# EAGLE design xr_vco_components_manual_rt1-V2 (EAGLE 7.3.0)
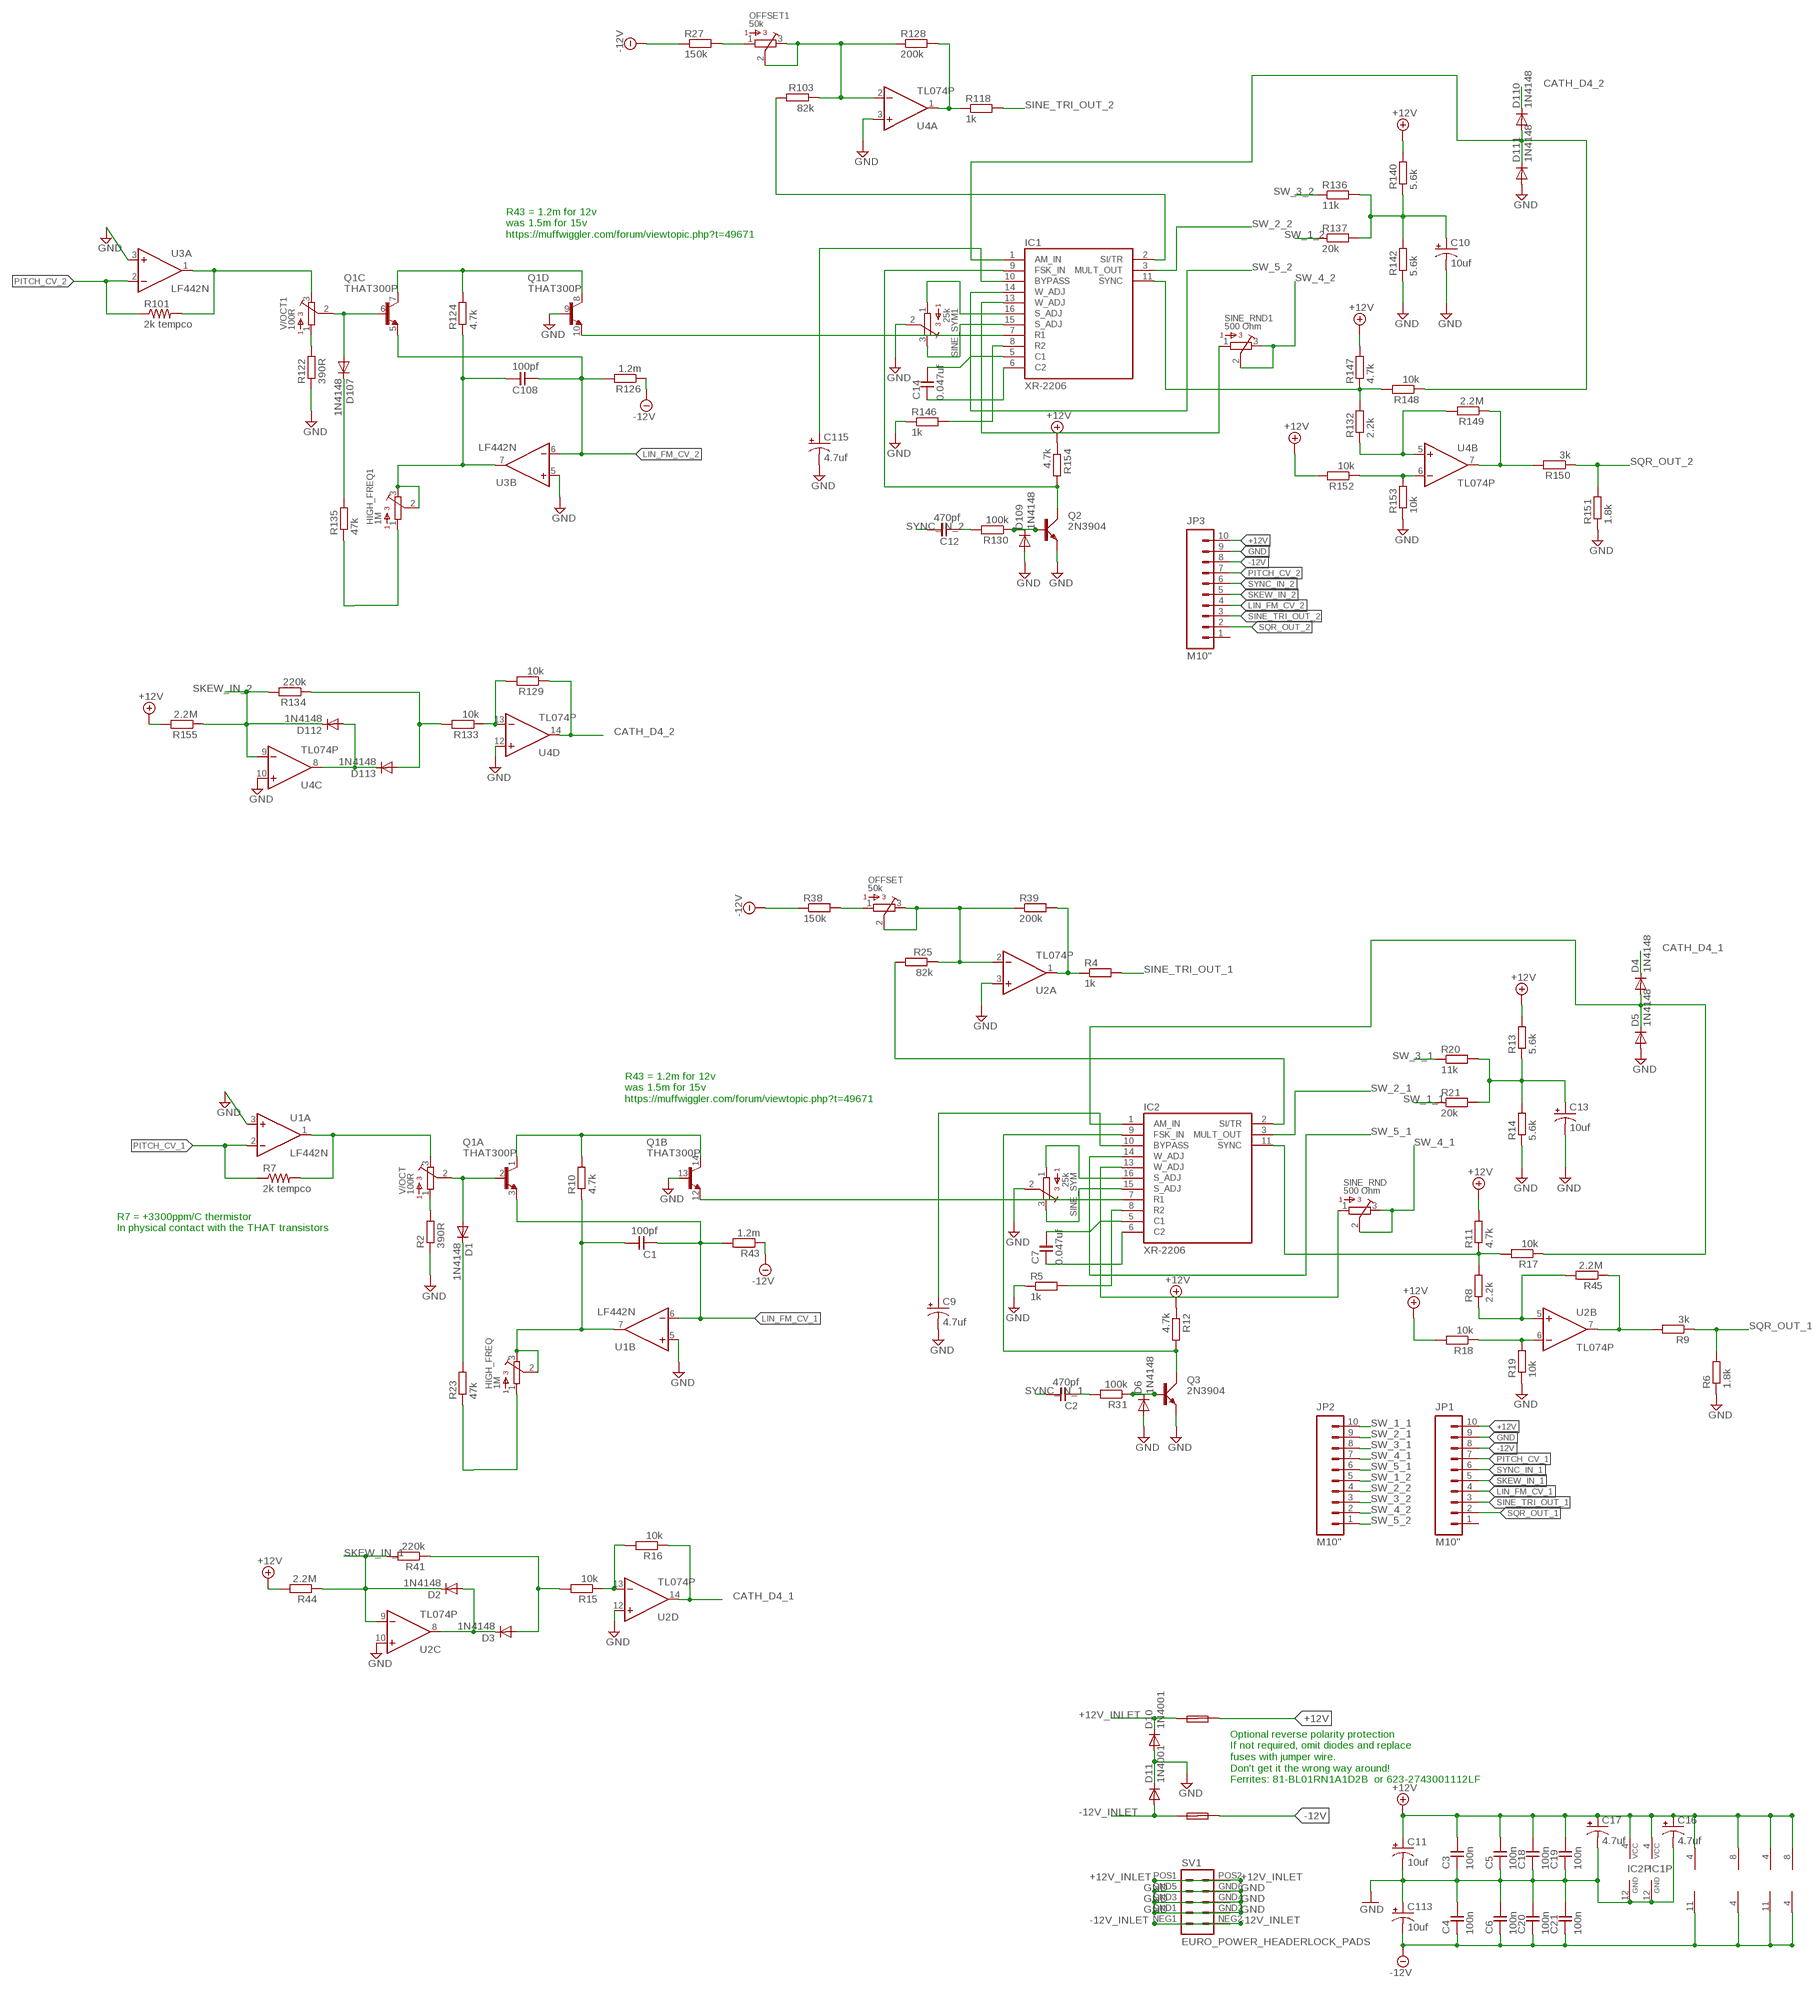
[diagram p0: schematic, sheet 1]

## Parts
C1  100pf  C-EU050-024X044  [C050-024X044]
C2  470pf  C-EU050-024X044  [C050-024X044]
C3  100n  C-EU050-024X044  [C050-024X044]
C4  100n  C-EU050-024X044  [C050-024X044]
C5  100n  C-EU050-024X044  [C050-024X044]
C6  100n  C-EU050-024X044  [C050-024X044]
C7  0.047uf  C-EU050-024X044  [C050-024X044]
C9  4.7uf  CAP_POLPTH2  [CPOL-RADIAL-10UF-25V]
C10  10uf  CAP_POLPTH2  [CPOL-RADIAL-10UF-25V]
C11  10uf  CAP_POLPTH2  [CPOL-RADIAL-10UF-25V]
C12  470pf  C-EU050-024X044  [C050-024X044]
C13  10uf  CAP_POLPTH2  [CPOL-RADIAL-10UF-25V]
C14  0.047uf  C-EU050-024X044  [C050-024X044]
C16  4.7uf  CAP_POLPTH2  [CPOL-RADIAL-10UF-25V]
C17  4.7uf  CAP_POLPTH2  [CPOL-RADIAL-10UF-25V]
C18  100n  C-EU050-024X044  [C050-024X044]
C19  100n  C-EU050-024X044  [C050-024X044]
C20  100n  C-EU050-024X044  [C050-024X044]
C21  100n  C-EU050-024X044  [C050-024X044]
C108  100pf  C-EU050-024X044  [C050-024X044]
C113  10uf  CAP_POLPTH2  [CPOL-RADIAL-10UF-25V]
C115  4.7uf  CAP_POLPTH2  [CPOL-RADIAL-10UF-25V]
D1  1N4148  SMALL_DIODEDO35-7  [DO35-7]
D2  1N4148  SMALL_DIODEDO35-7  [DO35-7]
D3  1N4148  SMALL_DIODEDO35-7  [DO35-7]
D4  1N4148  SMALL_DIODEDO35-7  [DO35-7]
D5  1N4148  SMALL_DIODEDO35-7  [DO35-7]
D6  1N4148  SMALL_DIODEDO35-7  [DO35-7]
D10  1N4001  1N4004  [DO41-10]
D11  1N4001  1N4004  [DO41-10]
D107  1N4148  SMALL_DIODEDO35-7  [DO35-7]
D109  1N4148  SMALL_DIODEDO35-7  [DO35-7]
D110  1N4148  SMALL_DIODEDO35-7  [DO35-7]
D111  1N4148  SMALL_DIODEDO35-7  [DO35-7]
D112  1N4148  SMALL_DIODEDO35-7  [DO35-7]
D113  1N4148  SMALL_DIODEDO35-7  [DO35-7]
F1  FUSE  PTC_FUSEPOLY_FUSE  [C050H075X075]
F2  FUSE  PTC_FUSEPOLY_FUSE  [C050H075X075]
HIGH_FREQ  1M  BOURNS_3362P_TRIMMERP  [BOURNS_3362P_TRIMMER]
HIGH_FREQ1  1M  BOURNS_3362P_TRIMMERP  [BOURNS_3362P_TRIMMER]
IC1  XR-2206  [DIL16]
IC2  XR-2206  [DIL16]
JP1  M10"  [1X10]
JP2  M10"  [1X10]
JP3  M10"  [1X10]
OFFSET  50k  BOURNS_3362P_TRIMMERP  [BOURNS_3362P_TRIMMER]
OFFSET1  50k  BOURNS_3362P_TRIMMERP  [BOURNS_3362P_TRIMMER]
Q1  THAT300P  [DIL14]
Q2  2N3904  [TO92D]
Q3  2N3904  [TO92D]
R2  390R  RESISTOR7MM  [7MM_RESISTOR]
R4  1k  RESISTOR7MM  [7MM_RESISTOR]
R5  1k  RESISTOR7MM  [7MM_RESISTOR]
R6  1.8k  RESISTOR7MM  [7MM_RESISTOR]
R7  2k tempco  R-US_0309/12  [0309/12]
R8  2.2k  RESISTOR7MM  [7MM_RESISTOR]
R9  3k  RESISTOR7MM  [7MM_RESISTOR]
R10  4.7k  RESISTOR7MM  [7MM_RESISTOR]
R11  4.7k  RESISTOR7MM  [7MM_RESISTOR]
R12  4.7k  RESISTOR7MM  [7MM_RESISTOR]
R13  5.6k  RESISTOR7MM  [7MM_RESISTOR]
R14  5.6k  RESISTOR7MM  [7MM_RESISTOR]
R15  10k  RESISTOR7MM  [7MM_RESISTOR]
R16  10k  RESISTOR7MM  [7MM_RESISTOR]
R17  10k  RESISTOR7MM  [7MM_RESISTOR]
R18  10k  RESISTOR7MM  [7MM_RESISTOR]
R19  10k  RESISTOR7MM  [7MM_RESISTOR]
R20  11k  RESISTOR7MM  [7MM_RESISTOR]
R21  20k  RESISTOR7MM  [7MM_RESISTOR]
R23  47k  RESISTOR7MM  [7MM_RESISTOR]
R25  82k  RESISTOR7MM  [7MM_RESISTOR]
R27  150k  RESISTOR7MM  [7MM_RESISTOR]
R31  100k  RESISTOR7MM  [7MM_RESISTOR]
R38  150k  RESISTOR7MM  [7MM_RESISTOR]
R39  200k  RESISTOR7MM  [7MM_RESISTOR]
R41  220k  RESISTOR7MM  [7MM_RESISTOR]
R43  1.2m  RESISTOR7MM  [7MM_RESISTOR]
R44  2.2M  RESISTOR7MM  [7MM_RESISTOR]
R45  2.2M  RESISTOR7MM  [7MM_RESISTOR]
R101  2k tempco  R-US_0309/12  [0309/12]
R103  82k  RESISTOR7MM  [7MM_RESISTOR]
R118  1k  RESISTOR7MM  [7MM_RESISTOR]
R122  390R  RESISTOR7MM  [7MM_RESISTOR]
R124  4.7k  RESISTOR7MM  [7MM_RESISTOR]
R126  1.2m  RESISTOR7MM  [7MM_RESISTOR]
R128  200k  RESISTOR7MM  [7MM_RESISTOR]
R129  10k  RESISTOR7MM  [7MM_RESISTOR]
R130  100k  RESISTOR7MM  [7MM_RESISTOR]
R132  2.2k  RESISTOR7MM  [7MM_RESISTOR]
R133  10k  RESISTOR7MM  [7MM_RESISTOR]
R134  220k  RESISTOR7MM  [7MM_RESISTOR]
R135  47k  RESISTOR7MM  [7MM_RESISTOR]
R136  11k  RESISTOR7MM  [7MM_RESISTOR]
R137  20k  RESISTOR7MM  [7MM_RESISTOR]
R140  5.6k  RESISTOR7MM  [7MM_RESISTOR]
R142  5.6k  RESISTOR7MM  [7MM_RESISTOR]
R146  1k  RESISTOR7MM  [7MM_RESISTOR]
R147  4.7k  RESISTOR7MM  [7MM_RESISTOR]
R148  10k  RESISTOR7MM  [7MM_RESISTOR]
R149  2.2M  RESISTOR7MM  [7MM_RESISTOR]
R150  3k  RESISTOR7MM  [7MM_RESISTOR]
R151  1.8k  RESISTOR7MM  [7MM_RESISTOR]
R152  10k  RESISTOR7MM  [7MM_RESISTOR]
R153  10k  RESISTOR7MM  [7MM_RESISTOR]
R154  4.7k  RESISTOR7MM  [7MM_RESISTOR]
R155  2.2M  RESISTOR7MM  [7MM_RESISTOR]
SINE_RND  500 Ohm  BOURNS_3362P_TRIMMERP  [BOURNS_3362P_TRIMMER]
SINE_RND1  500 Ohm  BOURNS_3362P_TRIMMERP  [BOURNS_3362P_TRIMMER]
SINE_SYM  25k  BOURNS_3362P_TRIMMERP  [BOURNS_3362P_TRIMMER]
SINE_SYM1  25k  BOURNS_3362P_TRIMMERP  [BOURNS_3362P_TRIMMER]
SV1  EURO_POWER_HEADERLOCK_PADS  [EURO_PWR_HEADER_LOCK]
U1  LF442N  [DIL08]
U2  TL074P  [DIL14]
U3  LF442N  [DIL08]
U4  TL074P  [DIL14]
V/OCT  100R  BOURNS_3362P_TRIMMERP  [BOURNS_3362P_TRIMMER]
V/OCT1  100R  BOURNS_3362P_TRIMMERP  [BOURNS_3362P_TRIMMER]

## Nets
+12V: C3.1 C5.1 C11.1(+) C16.1(+) C17.1(+) C18.1 C19.1 F1.2 IC1.4(VCC) IC2.4(VCC) JP1.10 JP3.10 R11.2 R12.1 R13.2 R18.2 R44.2 R140.2 R147.2 R152.2 R154.1 R155.2 U1.8(P:V+) U2.4(P:V+) U3.8(P:V+) U4.4(P:V+)
+12V_INLET [power]: D10.C F1.1 SV1.POS1 SV1.POS2
-12V: C4.2 C6.2 C20.2 C21.2 C113.2(-) F2.2 JP1.8 JP3.8 R27.1 R38.1 R43.1 R126.1 U1.4(P:V-) U2.11(P:V-) U3.4(P:V-) U4.11(P:V-)
-12V_INLET [power]: D11.A F2.1 SV1.NEG1 SV1.NEG2
CATH_D4_1: D4.C R16.1 U2.14(D:OUT)
CATH_D4_2: D110.C R129.1 U4.14(D:OUT)
GND: C3.2 C4.1 C5.2 C6.1 C9.2(-) C10.2(-) C11.2(-) C13.2(-) C16.2(-) C17.2(-) C18.2 C19.2 C20.1 C21.1 C113.1(+) C115.2(-) D5.A D6.A D10.A D11.C D109.A D111.A IC1.12(GND) IC2.12(GND) JP1.9 JP3.9 Q1.9(D:B) Q1.13(B:B) Q2.E Q3.E R2.1 R5.1 R6.1 R14.1 R19.1 R122.1 R142.1 R146.1 R151.1 R153.1 SINE_SYM1.2 SINE_SYM.2 SV1.GND1 SV1.GND2 SV1.GND3 SV1.GND4 SV1.GND5 SV1.GND6 U1.3(A:+IN) U1.5(B:+IN) U2.3(A:+IN) U2.10(C:+IN) U2.12(D:+IN) U3.3(A:+IN) U3.5(B:+IN) U4.3(A:+IN) U4.10(C:+IN) U4.12(D:+IN)
LIN_FM_CV_1: C1.2 JP1.4 Q1.3(A:E) R43.2 U1.6(B:-IN)
LIN_FM_CV_2: C108.2 JP3.4 Q1.5(C:E) R126.2 U3.6(B:-IN)
N$1: IC2.7(R1) Q1.12(B:E)
N$2: D1.C R23.2
N$3: HIGH_FREQ.1 R23.1
N$4: R101.2 U3.1(A:OUT) V/OCT1.3
N$5: IC2.2(SI/TR) R25.2
N$6: R122.2 V/OCT1.1
N$7: R7.2 U1.1(A:OUT) V/OCT.3
N$8: OFFSET.2 OFFSET.3 R25.1 R39.1 U2.2(A:-IN)
N$9: R2.2 V/OCT.1
N$10: D1.A Q1.2(A:B) V/OCT.2
N$11: Q1.1(A:C) Q1.14(B:C) R10.2
N$12: OFFSET.1 R38.2
N$13: R4.1 R39.2 U2.1(A:OUT)
N$14: D107.A Q1.6(C:B) V/OCT1.2
N$15: C1.1 HIGH_FREQ.2 HIGH_FREQ.3 R10.1 U1.7(B:OUT)
N$16: C13.1(+) R13.1 R14.2 R20.2 R21.2
N$17: IC2.16(S_ADJ) SINE_SYM.1
N$18: Q1.7(C:C) Q1.8(D:C) R124.2
N$19: C108.1 HIGH_FREQ1.2 HIGH_FREQ1.3 R124.1 U3.7(B:OUT)
N$20: IC2.13(W_ADJ) SINE_RND.1
N$21: IC2.15(S_ADJ) SINE_SYM.3
N$22: IC2.8(R2) R5.2
N$23: R18.1 R19.2 U2.6(B:-IN)
N$24: R9.2 R45.1 U2.7(B:OUT)
N$25: R15.1 R16.2 U2.13(D:-IN)
N$26: R8.1 R45.2 U2.5(B:+IN)
N$27: D4.A D5.C IC2.1(AM_IN) R17.1
N$28: C2.2 R31.2
N$29: D6.C Q3.B R31.1
N$30: IC2.11(SYNC) R8.2 R11.1 R17.2
N$31: IC2.9(FSK_IN) Q3.C R12.2
N$32: C7.2 IC2.6(C2)
N$33: C7.1 IC2.5(C1)
N$34: C9.1(+) IC2.10(BYPASS)
N$35: D2.A D3.C U2.8(C:OUT)
N$36: D3.A R15.2 R41.1
N$37: IC1.7(R1) Q1.10(D:E)
N$38: HIGH_FREQ1.1 R135.1
N$39: D107.C R135.2
N$40: IC1.2(SI/TR) R103.2
N$41: OFFSET1.2 OFFSET1.3 R103.1 R128.1 U4.2(A:-IN)
N$42: OFFSET1.1 R27.2
N$43: R118.1 R128.2 U4.1(A:OUT)
N$44: C10.1(+) R136.2 R137.2 R140.1 R142.2
N$45: IC1.13(W_ADJ) SINE_RND1.1
N$46: IC1.16(S_ADJ) SINE_SYM1.1
N$47: IC1.15(S_ADJ) SINE_SYM1.3
N$48: IC1.8(R2) R146.2
N$49: R152.1 R153.2 U4.6(B:-IN)
N$50: R149.1 R150.2 U4.7(B:OUT)
N$51: R132.1 R149.2 U4.5(B:+IN)
N$52: IC1.11(SYNC) R132.2 R147.1 R148.2
N$53: D110.A D111.C IC1.1(AM_IN) R148.1
N$54: C12.2 R130.2
N$55: D109.C Q2.B R130.1
N$56: IC1.9(FSK_IN) Q2.C R154.2
N$57: C14.2 IC1.6(C2)
N$58: C14.1 IC1.5(C1)
N$59: R129.2 R133.1 U4.13(D:-IN)
N$60: D112.A D113.C U4.8(C:OUT)
N$61: D113.A R133.2 R134.1
N$62: C115.1(+) IC1.10(BYPASS)
PITCH_CV_1: JP1.7 R7.1 U1.2(A:-IN)
PITCH_CV_2: JP3.7 R101.1 U3.2(A:-IN)
SINE_TRI_OUT_1: JP1.3 R4.2
SINE_TRI_OUT_2: JP3.3 R118.2
SKEW_IN_1: D2.C JP1.5 R41.2 R44.1 U2.9(C:-IN)
SKEW_IN_2: D112.C JP3.5 R134.2 R155.1 U4.9(C:-IN)
SQR_OUT_1: JP1.2 R6.2 R9.1
SQR_OUT_2: JP3.2 R150.1 R151.2
SW_1_1: JP2.10 R21.1
SW_1_2: JP2.5 R137.1
SW_2_1: IC2.3(MULT_OUT) JP2.9
SW_2_2: IC1.3(MULT_OUT) JP2.4
SW_3_1: JP2.8 R20.1
SW_3_2: JP2.3 R136.1
SW_4_1: JP2.7 SINE_RND.2 SINE_RND.3
SW_4_2: JP2.2 SINE_RND1.2 SINE_RND1.3
SW_5_1: IC2.14(W_ADJ) JP2.6
SW_5_2: IC1.14(W_ADJ) JP2.1
SYNC_IN_1: C2.1 JP1.6
SYNC_IN_2: C12.1 JP3.6
Unconnected: JP1.1 JP3.1

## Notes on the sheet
- R43 = 1.2m for 12v
  was 1.5m for 15v
  https://muffwiggler.com/forum/viewtopic.php?t=49671
- R43 = 1.2m for 12v
  was 1.5m for 15v
  https://muffwiggler.com/forum/viewtopic.php?t=49671
- R7 = +3300ppm/C thermistor
  In physical contact with the THAT transistors
- Optional reverse polarity protection
  If not required, omit diodes and replace
  fuses with jumper wire. 
  Don't get it the wrong way around! 
  Ferrites: 81-BL01RN1A1D2B  or 623-2743001112LF

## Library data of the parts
C1-C7 C12 C14 C18-C21 C108 = TomW:C-EU: CAPACITOR, European symbol
C9-C11 C13 C16 C17 C113 C115 = SparkFun-Passives:CAP_POL: Capacitor Polarized
D1-D6 D107 D109-D113 = MusicThingModular:SMALL_DIODE: Small Signal Diode
D10 D11 = diode:1N4004: DIODE
F1 F2 = TomW:PTC_FUSE
HIGH_FREQ HIGH_FREQ1 OFFSET OFFSET1 SINE_RND SINE_RND1 SINE_SYM SINE_SYM1 V/OCT V/OCT1 = MusicThingModular:BOURNS_3362P_TRIMMER: 3362 Series 1/4" Square Trimmer
IC1 IC2 = exar:XR-2206: Monolithic FUNCTION GENERATOR; OC_FARNELL: unknown; OC_NEWARK: unknown
JP1-JP3 = SparkFun-Connectors:M10: Header 10 Standard 10-pin 0.1" header. Use with straight break away headers (SKU : PRT-00116), right angle break away headers (PRT-00553), swiss pins (PRT-00743), machine pins (PRT-00117), and female headers (PRT-00115).
Q1 = that-corp:THAT300: 4-Matched NPN Transistors
Q2 Q3 = transistor-small-signal:2N3904: NPN TRANSISTOR
R2 R4-R6 R8-R21 R23 R25 R27 R31 R38 R39 R41 R43-R45 R103 R118 R122 R124 R126 R128-R130 R132-R137 R140 R142 R146-R155 = MusicThingModular:RESISTOR: Standard resistor, various versions
R7 R101 = resistor:R-US_: RESISTOR, American symbol
SV1 = MusicThingModular:EURO_POWER_HEADER: Power Header 10 pin power header for Eurorack Power Supplies Variants with fatter pads for easier soldering, and the LOCK variant which has 5mil offset pins to hold the component in place before soldering
U1 U3 = linear:LF442: OP AMP
U2 U4 = linear:TL074: OP AMP

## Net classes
1 power: width 0.406 mm
2 ground: width 0.305 mm

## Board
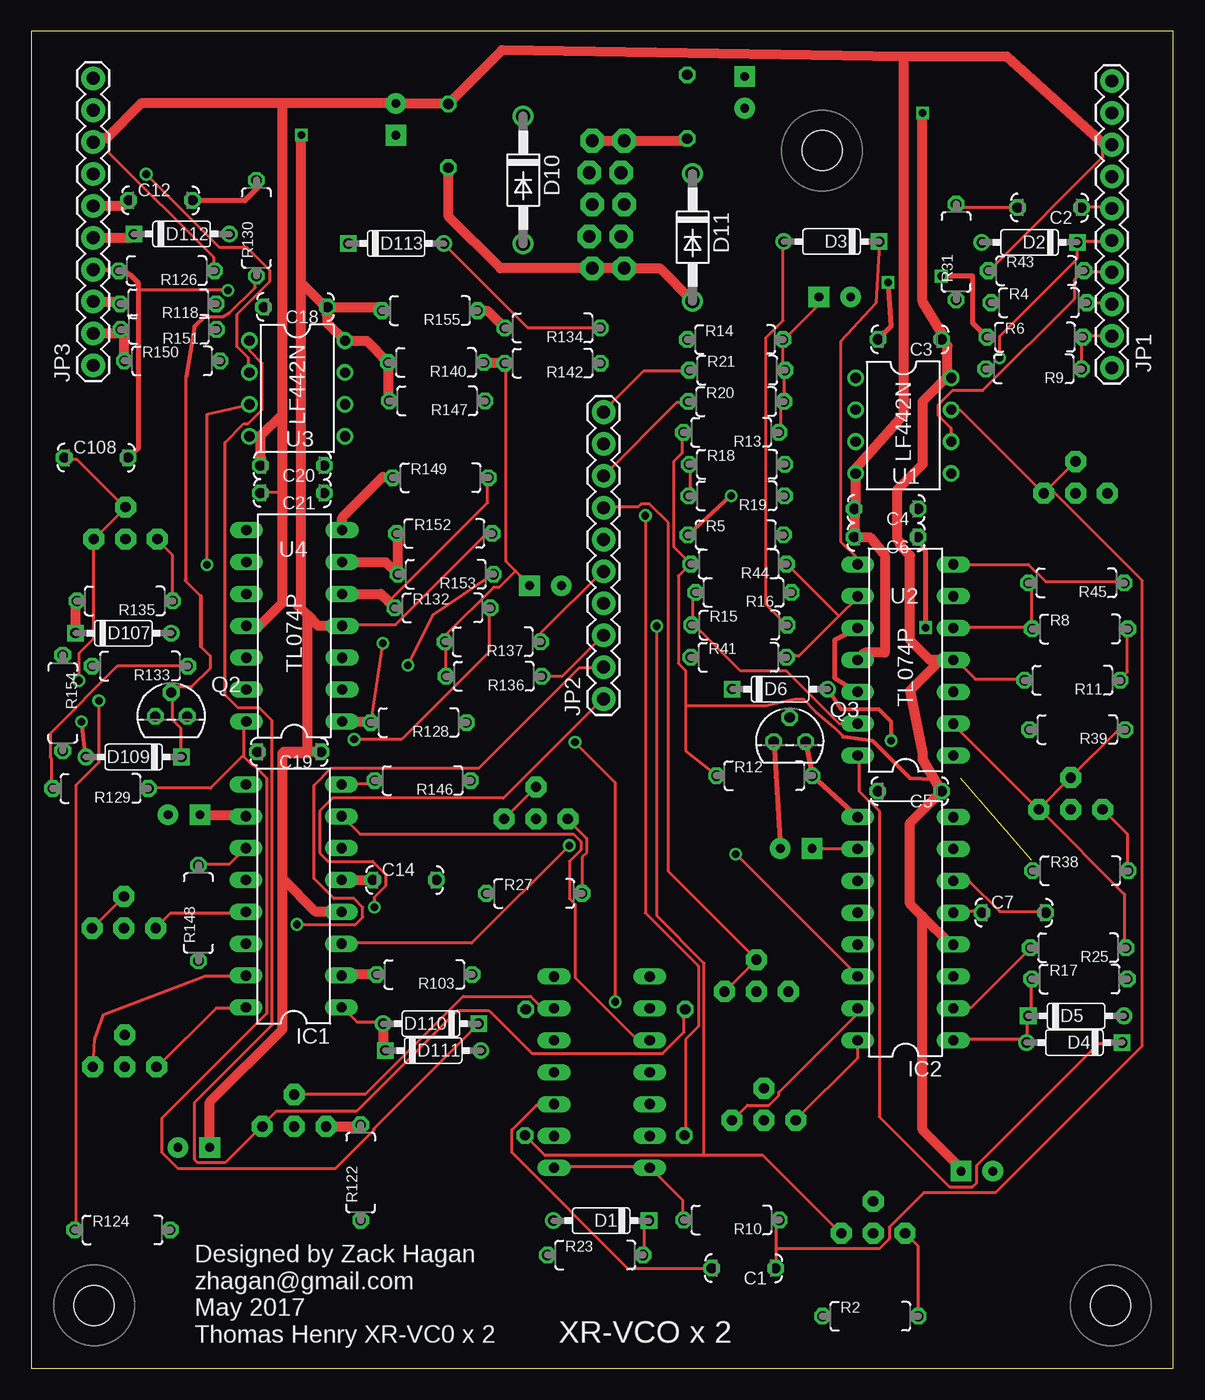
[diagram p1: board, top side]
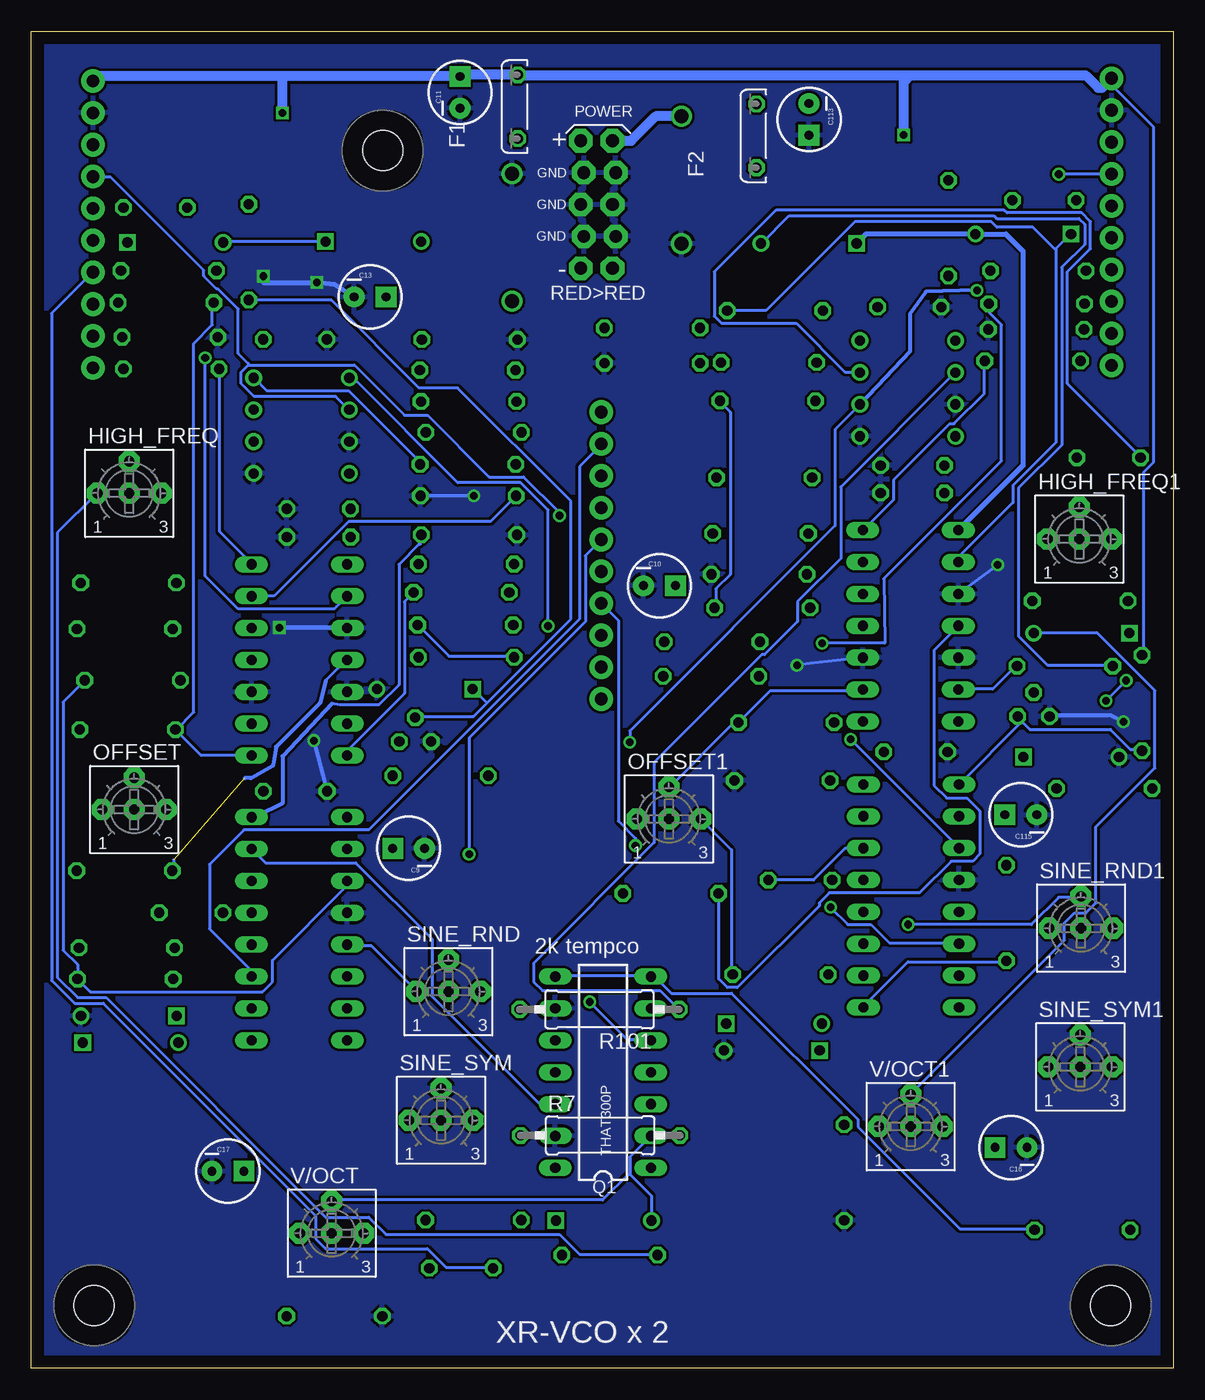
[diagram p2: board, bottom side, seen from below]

Size 91 x 106.5 mm. Coordinates in mm from the lower left corner, seen from the top.
Outline: 0,0 91,0 91,106.5 0,106.5 0,0
Copper layers (1*16): Top 0.035mm / dielectric 1.5mm / Bottom 0.035mm
Design rules "default *": minimum track width 10mil, minimum drill 19mil, track to track 8mil, track to pad 8mil, pad to pad 8mil, via to via 8mil, smd to smd 8mil, copper to edge 40mil, drill to drill 8mil, minimum pad ring 10mil, minimum via ring 8mil, stop-mask expansion 4mil, vias tented up to drill 0mil, thermal gap 10mil

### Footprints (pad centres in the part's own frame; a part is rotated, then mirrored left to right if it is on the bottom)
C050-024X044 = drill 0.813 octagon: 1 -2.54,0; 2 2.54,0
CPOL-RADIAL-10UF-25V = drill 0.7 pad 1.651 square: 1 1.27,0 | drill 0.7 pad 1.651: 2 -1.27,0
DO35-7 = drill 0.813: A 3.81,0 | drill 0.813 square: C -3.81,0
DO41-10 = drill 1.118: A 5.08,0; C -5.08,0
C050H075X075 = drill 0.813 octagon: 1 -2.54,0; 2 2.54,0
BOURNS_3362P_TRIMMER = drill 0.813 pad 1.676 octagon: 1 -2.54,0; 2 0,2.54; 3 2.54,0; 4 0,0
DIL16 = drill 0.813 long: 1 -8.89,-3.81; 2 -6.35,-3.81; 3 -3.81,-3.81; 4 -1.27,-3.81; 5 1.27,-3.81; 6 3.81,-3.81; 7 6.35,-3.81; 8 8.89,-3.81; 9 8.89,3.81; 10 6.35,3.81; 11 3.81,3.81; 12 1.27,3.81; 13 -1.27,3.81; 14 -3.81,3.81; 15 -6.35,3.81; 16 -8.89,3.81
1X10 = drill 1.016 pad 1.88: 1 0,0; 2 2.54,0; 3 5.08,0; 4 7.62,0; 5 10.16,0; 6 12.7,0; 7 15.24,0; 8 17.78,0; 9 20.32,0; 10 22.86,0
DIL14 = drill 0.813 long: 1 -7.62,-3.81; 2 -5.08,-3.81; 3 -2.54,-3.81; 4 0,-3.81; 5 2.54,-3.81; 6 5.08,-3.81; 7 7.62,-3.81; 8 7.62,3.81; 9 5.08,3.81; 10 2.54,3.81; 11 0,3.81; 12 -2.54,3.81; 13 -5.08,3.81; 14 -7.62,3.81
TO92D = drill 0.813 octagon: B 0,1.905; C 1.27,0; E -1.27,0
7MM_RESISTOR = drill 0.813 octagon: 1 -3.81,0; 2 3.81,0
0309/12 = drill 0.813 octagon: 1 -6.35,0; 2 6.35,0
EURO_PWR_HEADER_LOCK = drill 1.016 pad 1.88 octagon: GND1 -2.54,1.143; GND2 -2.54,-1.397; GND3 0,1.397; GND4 0,-1.143; GND5 2.54,1.143; GND6 2.54,-1.397; NEG1 -5.08,1.397; NEG2 -5.08,-1.143; POS1 5.08,1.397; POS2 5.08,-1.143
DIL08 = drill 0.813 pad 1.27: 1 -3.81,-3.81; 2 -1.27,-3.81; 3 1.27,-3.81; 4 3.81,-3.81; 5 3.81,3.81; 6 1.27,3.81; 7 -1.27,3.81; 8 -3.81,3.81
MOUNTING_HOLE = hole 3.2: 0,0

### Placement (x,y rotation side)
C1  56.75,7.96 180 top
C2  81.12,92.46 180 top
C3  69.99,81.96 180 top
C4  68.11,68.46 180 top
C5  69.98,45.96 180 top
C6  68.1,66.21 180 top
C7  78.28,36.29 0 top
C9  60.94,41.41 180 bottom
C10  40.96,62.34 0 bottom
C11  56.84,101.64 90 bottom
C12  10.29,93.04 0 top
C13  64.01,85.34 0 bottom
C14  29.74,38.89 0 top
C16  12.94,17.58 180 bottom
C17  75.34,15.69 0 bottom
C18  21.04,84.54 180 top
C19  20.54,49.1 180 top
C20  20.79,71.91 180 top
C21  20.79,69.72 180 top
C108  5.16,72.54 0 top
C113  29.04,99.49 270 bottom
C115  12.16,44.09 180 bottom
D1  45.4,11.75 180 top
D2  79.53,89.69 180 top
D3  63.75,89.75 180 top
D4  83.1,25.94 180 top
D5  83.24,28.06 0 top
D6  59.65,54.1 0 top
D10  39.19,94.65 270 top
D11  52.69,90.1 270 top
D107  7.33,58.56 0 top
D109  8.15,48.69 180 top
D110  31.83,27.44 180 top
D111  32.01,25.31 0 top
D112  11.97,90.35 0 top
D113  29.06,89.6 0 top
F1  52.25,100.5 90 bottom
F2  33.22,98.18 90 bottom
HIGH_FREQ  83.2,69.7 0 bottom
HIGH_FREQ1  7.5,66.05 0 bottom
IC1  20.9,37.62 90 top
IC2  69.65,35.01 90 top
JP1  86.09,79.69 90 top
JP2  45.59,53.31 90 top
JP3  4.93,79.9 90 top
OFFSET  82.81,44.5 0 bottom
OFFSET1  40.2,43.75 0 bottom
Q1  45.45,23.57 90 bottom
Q2  11.14,51.92 0 top
Q3  60.42,49.92 0 top
R2  66.85,4.14 0 top
R4  80.28,84.89 0 top
R5  56.12,66.39 0 top
R6  79.96,82.14 0 top
R7  45.68,18.54 0 bottom
R8  83.55,58.89 0 top
R9  79.86,79.61 180 top
R10  55.78,11.8 180 top
R11  82.94,54.8 180 top
R12  58.4,47.2 0 top
R13  55.76,74.55 180 top
R14  56.08,81.95 0 top
R15  56.42,59.2 0 top
R16  56.74,61.8 180 top
R17  83.51,31 0 top
R18  56.22,72.01 0 top
R19  56.19,69.49 180 top
R20  56.15,77.01 0 top
R21  56.24,79.51 0 top
R23  44.92,9.01 0 top
R25  83.4,33.49 180 top
R27  40.06,37.82 0 top
R31  73.68,88.92 90 top
R38  83.58,39.63 0 top
R39  83.33,50.87 180 top
R41  56.35,56.63 0 top
R43  80.06,87.44 0 top
R44  56.35,64.06 180 top
R45  83.26,62.56 180 top
R101  45.74,28.58 180 bottom
R103  31.31,31.36 180 top
R118  10.9,84.8 180 top
R122  26.24,15.58 90 top
R124  7.26,11.01 0 top
R126  10.78,87.43 180 top
R128  30.85,51.43 180 top
R129  5.51,46.18 180 top
R130  17.93,90.83 90 top
R132  32.76,60.57 0 top
R133  8.65,55.93 180 top
R134  41.53,82.87 180 top
R135  7.44,61.12 180 top
R136  36.85,55.12 180 top
R137  36.76,57.87 180 top
R140  32.24,80.12 180 top
R142  41.53,80.06 180 top
R146  31.17,46.81 180 top
R147  32.33,77.06 180 top
R148  13.31,36.26 90 top
R149  32.6,70.94 0 top
R150  11.22,80.25 0 top
R151  10.94,82.75 180 top
R152  32.9,66.5 0 top
R153  33.01,63.25 180 top
R154  2.5,53 270 top
R155  31.75,84.25 180 top
SINE_RND  57.77,30 0 bottom
SINE_RND1  7.37,35.05 0 bottom
SINE_SYM  58.36,19.75 0 bottom
SINE_SYM1  7.43,24 0 bottom
SV1  45.84,92.71 90 bottom
U1  69.48,75.09 270 top
U2  69.65,56.42 90 top
U3  21.18,78.05 270 top
U4  20.95,59.14 90 top
U$1  [MOUNTING_HOLE]  63,97 0 top
U$2  [MOUNTING_HOLE]  5,5 0 top
U$3  [MOUNTING_HOLE]  86,5 0 top
V/OCT  67.07,10.75 0 bottom
V/OCT1  20.94,19.25 0 bottom

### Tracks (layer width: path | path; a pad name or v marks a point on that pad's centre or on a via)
+12V  (via drill 0.6)
  Top 0.254: 52.12,52.76 52.12,55.58 51.55,56.15 51.55,63.12 52.46,64.04 R44.2 52.46,64.15 51.21,65.41 51.21,72.27 51.89,72.95 51.89,74.44 R13.2 | 52.12,52.76 52.12,49.18 R12.1 | R152.2 36.69,66.44 36.23,66.44 29.03,59.24 25.15,59.24 U4.4 | R11.2 79.1,54.89 75.21,54.89 73.84,56.26 U2.4 | 52.12,52.76 58.53,52.76 60.76,53.28 61.54,53.28 62.52,52.26 64.01,51.01 64.69,50.32
  Top 0.305: 64.69,50.32 67,50 70,47 71.92,46.95
  Top 0.813: C18.1 23.46,84.54 21.5,86.5 | 21.5,86.5 v21.5,98.25 | U4.4 22.86,59.14 22,60 | 22,60 21.5,60.5 | 21.25,60.75 21.5,60.5 | 21.5,60.5 21.5,86.5 | IC1.4 22.65,36.35 20,39 | 20,39 20,49 | C18.1 23.58,83.27 U3.8 26.69,81.86 R140.2 28.43,77.15 R147.2 | C18.1 27.65,84.54 R155.2 | C19.1 20.1,49.1 20,49 | C16.1 14.21,21.21 20,27 20,39 | U1.8 73.1,78.9 73,79 | 73,79 73,81.43 C3.1 72.53,82.47 71,85 v71,100 | 73,79 71,77 71,72 69,70 69,66 69.25,65.75 69.25,65.5 70,64.75 70,58 71.58,56.42 U2.4 72.42,56.42 70,54 71,49 71,48.48 71.92,46.95 C5.1 70,43.44 70,37 71,36 | IC2.4 73.26,33.74 71,36 | C17.1 74.07,15.93 71,19 71,36 | 20,49 22,49 22,60
  Bottom 0.254: R154.1 2.4,56.84 2.4,71.35 1.6,72.15 1.6,98.9 4.92,102.21 JP3.10 | R18.2 60.12,72.04 60.12,72.27 65.72,77.87 72.24,77.87 73.27,78.9 U1.8
  Bottom 0.813: 21,103 52,103 52.04,103.04 F1.2 56.71,103.04 C11.1 71,102.91 | 21,103 7,103 6,102 5.69,102 JP3.10 | 71,102.91 85.73,102.91 JP1.10 | v21.5,98.25 21.5,102.5 21,103 | v71,100 71,102.91
+12V_INLET
  Top 0.813: SV1.POS2 SV1.POS1 52.08,97.79 F1.1
  Bottom 0.813: SV1.POS2 43.21,97.79 41.27,99.73 D10.C | 52.08,97.79 F1.1
-12V  (1 unrouted)
  Top 0.254: 20,69.75 18.29,69.75 C21.2 | JP1.8 85.38,97.07 85.38,96.5 76.35,87.47 R43.1 | R126.1 14.52,87.47 14.52,88.5 6.17,96.84 6.17,97.64 6,98
  Top 0.813: 20,100.76 C113.2 29.08,100.72 F2.2 37.5,105 69.5,104.5 | 20,100.76 8.76,100.76 6,98 5.25,98 JP3.8 | JP1.8 85.53,97.47 77.75,104.5 69.5,104.5 | U3.4 18,74.24 | 18,74.24 18.24,74.24 20,76 | 20,76 20,100.76 | C20.2 18.25,73.99 18,74.24 | U4.11 18.14,59.14 20,61 20,69.75 20,76 | 69.5,104.5 69.5,76 65.67,71.67 U1.4 65.67,68.56 C4.2 C6.2 66.79,66.21 68,64.75 68,57 66.42,57 U2.11
  Bottom 0.254: R27.1 36.23,37.75 36.23,31 35.55,30.32 34.75,30.32 28.23,36.83 28.23,37.06 27.43,37.86 20.23,37.86 17.72,40.38 16,40.38 15.43,40.95 15.43,44.38 16.46,45.41 18.06,45.41 19.09,46.43 19.09,57.18 17.14,59.12 U4.11 | 79.67,40.49 79.67,39.69 R38.1 | 67.55,54.78 65.95,56.38 U2.11
  Bottom 0.305: 67.55,54.78 68,53 71.5,49.5 71.75,48 73.5,47 74,47
-12V_INLET
  Top 0.813: D11.A 50.08,87.63 SV1.NEG1 SV1.NEG2 37.37,87.63 33.25,91.75 33.25,95.61 F2.1
CATH_D4_1
  Top 0.254: D4.C 86.87,25.86 85.04,25.86 75.32,16.14 75.32,14.77 74.98,14.43 73.15,14.43 67.55,20.03 67.55,44.38 65.95,45.98 65.95,48.72 U2.14
  Bottom 0.254: U2.14 65.84,48.84 65.84,49.18 61.27,53.75 61.27,61.06 60.58,61.75 R16.1
CATH_D4_2
  Top 0.254: 16.92,48.72 17.6,48.03 17.72,48.03 18.75,47.01 18.75,28.26 10.4,19.92 10.4,17.17 11.66,15.92 24.23,15.92 27.32,19 27.32,19.12 35.55,27.35 D110.C | 16.92,48.72 16.92,51.35 17.03,51.46 U4.14 | R129.1 9.37,46.21 14.29,46.21 16.8,48.72 16.92,48.72
GND  (via drill 0.6)
  Top 0.254: v14,64 14,76 U3.3 | v30,56 32,60 R153.1
  Top 0.305: D6.A 64.5,52.5 67.5,52.5 68.5,51.5 v68.5,50 | R5.1 v55.75,69.5 | D109.A v4,51.5
  Top 0.406: v68.25,86.5 68.5,83.01 C3.2 | R6.1 76.11,82.14 75,83.25 75,87 v72.5,87 | v71.25,59 71.25,65 C6.1 | U2.10 64,58 64,55 U2.12 | Q3.E C9.2
  Bottom 0.254: SV1.GND1 46.98,90.21 46.93,90.22 | 44.58,90.21 SV1.GND2 | U4.10 v14,64 | U4.3 v30,56
  Bottom 0.305: v68.5,50 C5.2 | v55.75,69.5 R19.1 | v4,51.5 5,52 10,52
  Bottom 0.406: C13.2 66.84,86.34 v68.25,86.5 72.5,86.5 v72.5,87 | U2.10 v71.25,59
  pour Bottom: -3,111 -3,-2 95,-2 95,-1 95,111
LIN_FM_CV_1
  Top 0.254: Q1.3 41.6,20.95 40.23,20.95 38.29,19 38.29,17.17 47.55,7.92 54.18,7.92 C1.2 | U1.6 73.27,73.87 73.27,74.89 72.24,75.92 72.24,76.72 73.38,77.87 75.78,77.87 83.1,85.18 83.1,86.67 83.78,87.35 R43.2 83.9,87.35 86.07,87.35 JP1.4
  Bottom 0.254: C1.2 54.29,8.03 57.95,8.03 59.44,9.52 67.55,9.52 68.35,10.32 68.35,12.14 85.27,29.06 87.55,29.06 89.38,30.89 89.38,84.04 86.18,87.24 JP1.4
LIN_FM_CV_2  (via drill 0.61)
  Top 0.254: v46.52,29.18 46.52,46.66 v43.32,49.86 | v15.66,85.87 8.5,85.87
  Top 0.406: JP3.4 R126.2 arc-40 8,87 8.5,86.5 8.5,85.87 8.5,73.25 C108.2
  Bottom 0.254: v46.52,29.18 43.55,26.2 41.72,26.2 Q1.5 | v43.32,49.86 43.32,50.78 26.98,67.12 26.98,74.78 25.03,76.72 U3.6 24.92,76.84 24.69,76.84
  Bottom 0.305: v15.66,85.87 19.75,85.75 21,84 21,81 U3.6
N$1
  Bottom 0.254: Q1.12 49.26,21.06 50.52,21.06 59.09,29.63 59.09,34.2 65.15,40.26 72.35,40.26 73.38,41.29 IC2.7
N$2
  Top 0.254: R23.2 48.81,9.06 48.81,11.34 49.15,11.69 D1.C
N$3
  Bottom 0.254: R23.1 41.15,9.06 47.32,9.06 48.92,10.66 62.75,10.66 64.12,12.03 67.55,12.03 85.04,29.52 87.33,29.52 88.92,31.12 88.92,66.55 85.84,69.64 HIGH_FREQ.1
N$4
  Top 0.254: R101.2 52.01,28.49 52.01,26.77 50.29,25.06 39.89,25.06 36.46,28.49 33.95,28.49 25.95,20.49 19.55,20.49 18.4,19.34 V/OCT1.3 18.29,19.23 15.43,16.37 13.26,16.37 13.03,16.6 13.03,21.17 19.2,27.35 19.2,51.58 18.17,52.61 16.46,52.61 15.43,53.63 15.43,73.75 16.92,75.24 17.26,75.24 18.4,76.38 18.4,80.04 17.37,81.07 17.37,81.75 U3.1
N$5
  Top 0.254: IC2.2 73.5,28.72 74.87,28.72 79.55,33.4 R25.2
N$6
  Top 0.813: V/OCT1.1 26.1,19.25 R122.2
N$7  (via drill 0.61)
  Top 0.254: 53.61,16.95 58.29,16.95 64.47,10.77 V/OCT.3 | 53.61,16.95 40.92,16.95 39.43,18.43 R7.2 | v49.84,59.12 49.84,36.03 53.61,32.26 53.61,16.95
  Bottom 0.254: v49.84,59.12 49.84,68.38 52.01,70.55 57.04,70.55 65.38,78.9 65.61,78.9 U1.1
N$8
  Top 0.254: R39.1 87.1,50.78 86.53,50.78 82.87,47.12 OFFSET.2 82.75,47.01 80.35,44.61 OFFSET.3 | R25.1 87.1,33.52 87.1,37.75 80.35,44.49 OFFSET.3 | U2.2 73.5,51.23 80.24,44.49 OFFSET.3
N$9
  Top 0.254: R2.2 70.64,4.14 70.64,9.74 69.72,10.66 V/OCT.1
N$10
  Bottom 0.254: 43.32,15.46 41.6,13.74 41.6,11.8 D1.A | 43.32,15.46 43.32,16.83 41.72,18.43 Q1.2 | V/OCT.2 66.98,13.4 45.49,13.4 43.43,15.46 43.32,15.46
N$11
  Top 0.254: Q1.1 41.72,16.03 49.15,16.03 Q1.14 49.38,15.92 51.89,13.4 51.89,11.8 R10.2
N$12
  Top 0.254: R38.2 87.33,39.69 87.33,42.55 85.38,44.49 OFFSET.1
N$13
  Bottom 0.254: U2.1 73.5,48.84 77.5,48.84 79.44,50.78 R39.2 79.44,50.89 78.07,52.26 78.07,81.64 76.58,83.12 76.58,84.84 R4.1
N$14
  Top 0.254: Q1.6 41.6,28.72 40.69,28.72 39.78,29.63 34.4,29.63 26.63,21.86 21.03,21.86 V/OCT1.2
  Bottom 0.254: D107.A 11.09,58.55 6.06,58.55 1.49,53.98 1.49,47.81 6.17,43.12 6.17,37.06 6.97,36.26 7.89,36.26 8.69,35.46 8.69,34.09 20.92,21.86 V/OCT1.2
N$15
  Top 0.254: 59.32,9.52 59.32,11.46 59.55,11.69 R10.1 | 59.32,9.52 59.32,8.03 C1.1 | U1.7 73.38,76.27 74.07,76.27 80.58,69.75 HIGH_FREQ.3 | HIGH_FREQ.2 83.1,72.15 80.7,69.75 HIGH_FREQ.3 | 59.32,9.52 67.55,9.52 68.35,10.32 68.35,11.23 71.09,13.97 76.81,13.97 88.47,25.63 88.47,62.78 81.15,70.09 HIGH_FREQ.3
N$16
  Top 0.254: R13.1 59.66,74.55 59.66,76.72 59.89,76.95 R20.2 60.01,77.07 60.01,79.47 R21.2 59.89,79.47 59.89,81.87 R14.2 60.01,81.98 62.64,84.61 62.64,85.3 C13.1
N$17
  Top 0.254: IC2.16 65.84,26.09 65.84,24.72 60.92,19.8 SINE_SYM.1
N$18
  Bottom 0.254: R124.2 11.09,11.12 17.03,11.12 25.15,19.23 25.15,19.8 35.2,29.86 40.01,29.86 41.26,31.12 41.6,31.12 Q1.7 41.72,31.23 49.15,31.23 Q1.8
N$19  (via drill 0.61)
  Top 0.254: C108.1 2.97,72.38 3.66,72.38 7.43,68.61 HIGH_FREQ1.2 7.43,68.49 5.03,66.09 HIGH_FREQ1.3 4.92,65.98 4.92,58.09 3.77,56.95 v3.77,54.78 | v5.37,53.18 5.37,48.26 3.54,46.43 3.54,11.12 R124.1
  Top 0.813: 2.45,72.71 C108.1
  Bottom 0.254: U3.7 25.03,79.35 26.18,79.35 30.06,83.24 36.01,83.24 36.58,83.81 36.58,87.35 31.66,92.27 13.49,92.27 13.26,92.04 7.32,92.04 6.63,91.35 6.63,89.18 8.46,87.35 8.46,78.44 2.63,72.61 C108.1 | v3.77,54.78 v5.37,53.18
N$20
  Bottom 0.254: IC2.13 65.84,33.63 63.89,33.63 60.35,30.09 SINE_RND.1
N$21
  Top 0.254: IC2.15 65.84,28.6 65.84,28.26 59.55,21.97 59.55,21.75 58.75,20.95 57.04,20.95 55.89,19.8 SINE_SYM.3
N$22
  Bottom 0.254: R5.2 60.01,66.32 60.01,65.64 60.12,65.64 61.72,64.04 61.72,54.44 63.32,52.84 66.41,52.84 67.05,52.94
  Bottom 0.305: 67.05,52.94 71,48.75 71,45 73,44 IC2.8
N$23
  Top 0.254: R19.2 52.46,69.52 52.46,71.92 R18.1
  Bottom 0.254: U2.6 73.38,61.52 71.67,61.52 65.72,67.47 54.41,67.47 52.46,69.41 R19.2
N$24
  Top 0.254: R45.1 86.98,62.66 80.81,62.66 79.44,64.04 73.5,64.04 U2.7
  Bottom 0.254: R9.2 76.01,79.58 76.01,66.67 73.5,64.15 U2.7
N$25
  Top 0.254: R16.2 52.92,61.75 52.69,61.52 52.69,59.24 R15.1 52.81,59.24 56.46,55.58 60.12,55.58 64.35,51.35 U2.13
N$26
  Top 0.254: R45.2 79.55,62.55 79.67,62.44 79.67,58.89 R8.1 79.55,59.01 73.5,59.01 U2.5
N$27
  Top 0.254: IC2.1 73.5,26.2 79.21,26.2 D4.A 79.32,25.98 79.32,28.03 D5.C 79.44,28.15 79.67,28.38 79.67,30.89 R17.1
N$28
  Top 0.254: C2.2 78.52,92.5 73.95,92.5 73.72,92.73 R31.2
N$29
  Bottom 0.254: 54.69,53.01 55.78,51.92 60.35,51.92 Q3.B | 54.69,53.01 48.01,59.69 48.01,69.07 57.04,78.1 60.12,78.1 67.09,85.07 73.61,85.07 R31.1 | 54.69,53.01 55.78,54.09 D6.C
N$30
  Top 0.254: R8.2 87.33,58.78 87.33,55.46 86.75,54.89 R11.1
  Bottom 0.254: R11.1 86.75,54.78 88.47,53.06 88.47,33.29 87.33,32.15 R17.2 87.21,30.89 86.3,29.98 72.58,29.98 71.78,30.77 71.78,32.49 65.95,38.32 65.95,38.78 IC2.11
N$31
  Top 0.406: Q3.C R12.2 IC2.9
N$32
  Top 0.254: C7.2 80.81,36.38 77.15,36.38 74.75,38.78 73.5,38.78 IC2.6
N$33
  Top 0.254: IC2.5 73.5,36.38 75.67,36.38 C7.1
N$34
  Top 0.254: IC2.10 65.84,41.41 62.29,41.41 C9.1
N$35
  Top 0.254: U2.8 65.84,64.15 65.84,64.49 64.47,65.86 64.47,81.78 67.3,84.87 67.55,89.64 D3.C
  Bottom 0.254: D2.A 75.67,89.75 67.67,89.75 D3.C
N$36
  Top 0.254: D3.A 59.89,89.64 59.89,83.47 58.52,82.1 58.52,60.84 60.12,59.24 R15.2
  Bottom 0.254: R41.1 52.58,56.72 57.72,56.72 60.12,59.12 R15.2
N$37
  Top 0.254: Q1.10 49.15,26.2 48.23,26.2 43.32,31.12 43.32,36.95 42.86,37.41 42.86,40.38 43.78,41.29 43.78,41.98 43.2,42.55 26.18,42.55 24.8,43.92 IC1.7
N$38
  Top 0.254: R135.1 11.2,61.18 11.2,64.84 10.06,65.98 HIGH_FREQ1.1
N$39
  Top 0.813: D107.C 3.52,61.01 R135.2
N$40
  Top 0.813: R103.2 24.8,31.36 IC1.2
N$41
  Top 0.254: OFFSET1.3 37.72,43.81 40.12,46.21 OFFSET1.2
  Bottom 0.254: R103.1 35.2,31.46 35.2,41.29 37.6,43.69 OFFSET1.3 | OFFSET1.2 40.12,46.32 35.09,51.35 34.75,51.35 R128.1 34.63,51.46 32.12,53.98 24.8,53.98 U4.2
N$42
  Top 0.254: R27.2 43.89,37.86 43.89,40.72 44.23,41.06 44.23,42.2 42.75,43.69 OFFSET1.1
N$43  (via drill 0.6)
  Top 0.254: v28,57.75 R128.2
  Top 0.813: U4.1 26.95,51.52 R128.2
  Bottom 0.254: R118.1 14.63,84.72 14.63,84.04 13.72,83.12 13.72,72.27 23.09,62.89 23,57.75 v28,57.75 | 24.69,51.58 U4.1
N$44
  Top 0.254: R136.2 33.03,57.86 R137.2 33.03,57.98 33.03,58.44 36.8,62.21 37.26,62.21 38.58,63.52 | 38.58,63.52 39.66,62.44 C10.1 | 38.58,63.52 37.83,64.27 37.83,79.7 R142.2
  Top 0.813: R142.2 36.11,80.06 R140.1
N$45
  Top 0.254: IC1.13 17.03,36.26 11.09,36.26 9.94,35.12 SINE_RND1.1
N$46
  Top 0.254: IC1.16 17.03,28.72 14.74,28.72 10.06,24.03 SINE_SYM1.1
N$47
  Top 0.254: IC1.15 17.03,31.23 13.83,31.23 5.77,28.18 5.06,26.18 4.92,24.03 SINE_SYM1.3
N$48
  Top 0.254: IC1.8 24.8,46.55 27.09,46.55 27.32,46.78 R146.2
N$49
  Top 0.813: U4.6 28.23,64.22 R153.2 29.2,66.39 R152.1
N$50
  Top 0.813: U4.7 24.76,67.76 28,71 28.73,71 R149.1
  Bottom 0.254: R150.2 15.09,80.15 15.09,77.64 17.49,75.24 17.83,75.24 22.29,70.78 22.29,69.18 24.69,66.78 U4.7
N$51
  Top 0.254: 28.46,61.06 36.35,68.95 36.35,70.89 R149.2
  Top 0.813: U4.5 27.84,61.68 28.46,61.06 R132.1
N$52  (via drill 0.61)
  Top 0.254: R148.2 13.37,40.15 15.77,40.15 17.03,41.41 IC1.11 | v25.72,50.09 29.49,50.09 36.46,57.06 36.46,60.49 R132.2
  Bottom 0.254: R132.2 36.46,60.61 36.46,62.09 35.32,63.24 35.32,76.15 36.12,76.95 R147.1 | v25.72,50.09 17.14,41.52 IC1.11
N$53
  Top 0.254: D110.A 27.66,27.57 25.95,27.57 24.8,28.72 IC1.1
  Top 0.813: D110.A 28.02,25.49 D111.C
  Bottom 0.254: R148.1 13.37,32.38 21.14,32.38 24.69,28.83 IC1.1
N$54
  Top 0.406: C12.2 16.96,93.04 17,93 18,94 18,94.57 R130.2
N$55
  Top 0.254: 13.5,61.5 12.25,62.75 12.34,62.89 12.34,79.01 | 13.5,57.5 14.25,56.75 14.25,55.75 12.75,54.25 11.56,54.25 Q2.B 11.2,53.63 11.2,51.69 11.89,51.01 11.89,48.72 D109.C | R130.1 17.83,87.01 17.83,86.1 15.77,84.04 15.25,83.75 13.75,83.75
  Top 0.305: 13.5,61.5 13.5,57.5 | 13.75,83.75 13,83 12.34,79.01
N$56
  Bottom 0.254: R154.2 2.52,49.29 3.43,49.29 5.03,50.89 11.43,50.89 12.34,51.81 Q2.C 12.12,51.46 17.03,46.55 IC1.9
N$57
  Bottom 0.254: C14.2 32.23,38.89 28.69,38.89 26.18,41.41 24.8,41.41 IC1.6
N$58
  Top 0.813: IC1.5 C14.1
N$59
  Top 0.254: R129.2 1.6,46.21 1.6,48.61 1.49,48.72 1.49,50.55 6.86,55.92 R133.1
  Bottom 0.254: U4.13 17.03,54.09 14.4,54.09 12.57,55.92 R133.1
N$60
  Bottom 0.406: D113.C 24.5,90.35 D112.A 13.35,90.35 12,89 12,71.9 U4.8
N$61
  Top 0.254: R134.1 45.26,82.9 39.55,82.9 32.92,89.53 D113.A
  Bottom 0.254: R133.2 4.92,56.04 10.06,56.04 12.34,58.32 12.34,70.09 8.91,73.52 8.91,87.7 7.09,89.53 7.09,91.13 7.54,91.58 14.06,91.58 14.29,91.81 30.63,91.81 32.8,89.64 D113.A
N$62
  Top 0.813: C115.1 16.97,44.09 IC1.10
PITCH_CV_1  (via drill 0.61)
  Top 0.254: v48.92,67.92 48.92,36.26 53.15,32.03 53.15,27.23 52.12,26.2 52.12,18.55 R7.1
  Bottom 0.254: v48.92,67.92 48.92,68.15 51.78,71.01 54.52,71.01 59.44,75.92 61.27,75.92 65.27,79.92 73.72,79.92 | 73.72,79.92 74.3,79.35 74.3,78.44 73.27,77.41 66.75,77.41 65.72,76.38 U1.2 | JP1.7 86.07,94.9 84.7,94.9 77.27,87.47 77.27,87.01 76.24,85.98 76.12,85.98 74.52,84.38 74.52,80.84 73.72,80.04 73.72,79.92
PITCH_CV_2  (via drill 0.61)
  Top 0.254: v9.14,95.13 14.97,89.3 17.14,89.3 18.97,87.47 18.97,86.55 16.34,83.92 16.34,81.41 17.26,80.5 17.26,79.35 U3.2
  Bottom 0.254: v9.14,95.13 5.03,95.13 JP3.7 | R101.1 39.43,28.6 40.92,30.09 50.29,30.09 50.98,30.77 50.98,32.26 41.38,41.86 41.38,48.26 32.8,56.84 32.58,56.84 29.95,59.47 29.95,61.06 26.52,64.49 26.52,70.21 17.37,79.35 U3.2
SINE_TRI_OUT_1
  Top 0.254: R4.2 84.12,84.84 86.07,84.84 JP1.3
SINE_TRI_OUT_2
  Top 0.813: JP3.3 6.91,84.98 R118.2
SKEW_IN_1  (via drill 0.61)
  Top 0.254: JP1.5 86.07,89.75 83.44,89.75 D2.C 83.33,89.64 83.33,88.38 77.15,82.21 v77.15,80.5 | 64.35,59.92 65.84,61.41 U2.9 | 64.35,59.92 61.15,56.72 60.24,56.72 R41.2 | 64.35,59.92 60.24,64.04 R44.1
  Bottom 0.254: v77.15,80.5 77.15,63.12 74.52,60.49 66.86,60.49 65.95,61.41 U2.9
SKEW_IN_2
  Top 0.813: JP3.5 7.87,90.06 D112.C | R155.1 36.34,84.25 R134.2
  Bottom 0.254: 9.37,89.18 9.37,73.75 12.8,70.32 12.8,68.95 17.03,64.72 17.03,64.27 U4.9 | 9.37,89.18 8.23,90.33 D112.C | R155.1 35.55,84.27 32.46,84.27 25.38,91.35 14.52,91.35 14.06,90.9 11.2,90.9 9.49,89.18 9.37,89.18
SQR_OUT_1
  Top 0.254: R9.1 83.67,79.7 83.67,82.1 R6.2 83.78,82.21 86.07,82.21 JP1.2
SQR_OUT_2
  Top 0.813: JP3.2 6.82,82.44 R151.2 7.41,82.47 R150.1
SW_1_1
  Top 0.254: R21.1 52.35,79.47 48.81,79.47 45.61,76.27 JP2.10
SW_1_2
  Top 0.254: R137.1 40.58,57.98 40.58,58.55 45.49,63.47 JP2.5
SW_2_1
  Bottom 0.254: IC2.3 73.5,31.23 73.5,31.69 76.81,35.01 76.81,40.15 74.07,42.89 64.12,42.89 47.32,59.69 47.32,71.81 45.61,73.52 JP2.9
SW_2_2  (via drill 0.61)
  Top 0.254: v42.86,41.63 35.09,33.86 24.8,33.86 IC1.3
  Bottom 0.254: v42.86,41.63 42.86,42.2 44.23,43.58 44.23,59.58 45.49,60.84 JP2.4
SW_3_1
  Top 0.254: R20.1 52.23,76.95 51.44,76.95 45.61,71.12 JP2.8
SW_3_2
  Top 0.254: R136.1 40.69,55.12 42.29,55.12 45.49,58.32 JP2.3
SW_4_1
  Top 0.254: SINE_RND.3 55.32,30.09 57.72,32.49 SINE_RND.2 57.72,32.6 50.75,39.58 50.75,67.35 49.26,68.84 48.58,68.84 48.35,68.61 45.61,68.61 JP2.7
SW_4_2  (via drill 0.61)
  Top 0.254: SINE_RND1.3 4.92,35.12 7.32,37.52 SINE_RND1.2 | v21.14,35.35 25.83,35.35 26.4,35.92 26.4,36.72 25.72,37.41 24.12,37.41 22.52,39.01 22.52,46.43 23.89,47.81 35.66,47.81 43.66,55.81 45.49,55.81 JP2.2
  Bottom 0.254: v21.14,35.35 11.32,35.35 9.14,37.52 7.43,37.52 SINE_RND1.2
SW_5_1  (via drill 0.61)
  Top 0.254: v56.12,40.95 65.84,31.23 IC2.14
  Bottom 0.254: v56.12,40.95 56.12,50.21 46.86,59.47 46.86,64.72 45.61,65.98 JP2.6
SW_5_2  (via drill 0.61)
  Top 0.254: v27.32,36.72 27.32,37.52 28.23,38.43 28.23,39.35 27.2,40.38 23.66,40.38 22.97,41.06 22.97,44.38 24,45.41 37.6,45.41 45.49,53.29 JP2.1
  Bottom 0.254: v27.32,36.72 25.95,35.35 24.12,35.35 22.63,33.86 17.14,33.86 IC1.14
SYNC_IN_1
  Top 0.254: C2.1 83.67,92.5 86.07,92.5 JP1.6
SYNC_IN_2
  Top 0.813: JP3.6 7.31,92.6 C12.1

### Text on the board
tNames: Designed by Zack Hagan / zhagan@gmail.com / May 2017 / Thomas Henry XR-VC0 x 2 | XR-VCO x 2
bNames: XR-VCO x 2

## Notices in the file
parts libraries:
SparkFun-Passives: Licensing: CC v3.0 Share-Alike You are welcome to use this library for commercial purposes.
that-corp: Copyright (C) 2008-2010, Bob Starr
